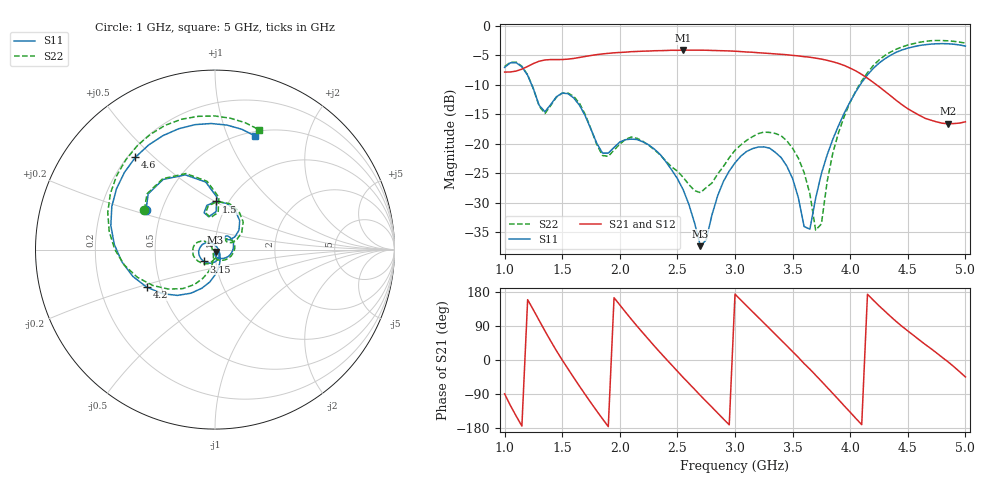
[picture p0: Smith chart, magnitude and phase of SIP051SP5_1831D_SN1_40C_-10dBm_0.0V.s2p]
# GHz  S  dB  R  50
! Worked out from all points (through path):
!   81 points, 1 GHz to 5 GHz, reference 50 ohm
!   highest |S21| = -4.14 dB at 2.55 GHz (marker M1); lowest = -16.6 dB at 4.85 GHz (marker M2)
!   lowest |S11| = -37.4 dB at 2.7 GHz (marker M3), VSWR 1.03, Z = 50.3 - j1.33 ohm
!   |S11| at or under -10 dB: 1.235 GHz to 4.087 GHz (2.853 GHz wide, 107 % of centre)
!   |S22| runs from -34.7 to -2.5 dB; largest |S21 - S12| = 0.0056
!   S11 on the Smith chart (normalised r, x): 1 GHz: 0.41, +0.23; 1.5 GHz: 0.87, +0.51; 3.15 GHz: 0.88, -0.12; 4.2 GHz: 0.42, -0.21; 4.6 GHz: 0.23, +0.44; 5 GHz: 0.54, +1.26
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1  -7.06 150.0  -7.86 -89.3  -7.85 -89.4  -6.91 150.7
1.15  -6.98 111.6  -7.36 -174.3  -7.37 -174.3  -6.86 110.9
1.3  -13.50 88.4  -6.02 104.4  -6.03 104.4  -13.63 85.2
1.5  -11.43 88.9  -5.74 0.1  -5.72 0.0  -11.44 86.7
1.7  -15.29 39.1  -5.21 -91.3  -5.22 -91.0  -15.06 32.6
1.95  -20.64 52.5  -4.59 164.4  -4.61 164.4  -21.09 43.4
2.15  -19.29 18.6  -4.37 89.3  -4.36 89.5  -19.09 4.6
2.35  -21.82 -30.5  -4.23 19.9  -4.22 19.7  -21.89 -45.7
2.55  -27.80 -80.8  -4.14 -46.1  -4.14 -45.8  -25.71 -81.5
2.7  -37.38 -78.1  -4.15 -93.7  -4.16 -93.7  -28.31 -89.4
3  -23.26 -90.0  -4.32 173.8  -4.33 173.7  -21.12 -116.5
3.15  -20.85 -133.1  -4.50 128.1  -4.51 128.1  -18.84 -145.8
3.3  -20.75 -175.0  -4.71 83.0  -4.71 82.8  -18.09 -175.5
3.5  -25.92 128.3  -5.03 22.1  -5.03 22.1  -20.78 149.2
3.6  -34.05 67.7  -5.24 -9.5  -5.24 -8.9  -24.89 134.9
3.7  -29.28 -39.2  -5.50 -40.0  -5.49 -39.8  -34.66 154.2
3.9  -16.89 -90.4  -6.41 -104.9  -6.42 -104.9  -18.06 -105.8
4.2  -7.25 -151.2  -9.61 158.0  -9.61 157.9  -6.77 -160.3
4.35  -5.01 177.1  -11.87 115.0  -11.89 115.0  -4.46 170.2
4.6  -3.36 130.7  -15.18 53.0  -15.23 53.0  -2.81 126.6
4.85  -3.06 91.8  -16.62 -4.9  -16.61 -5.4  -2.56 90.1
5  -3.45 70.8  -16.29 -44.6  -16.31 -44.8  -2.96 69.9
